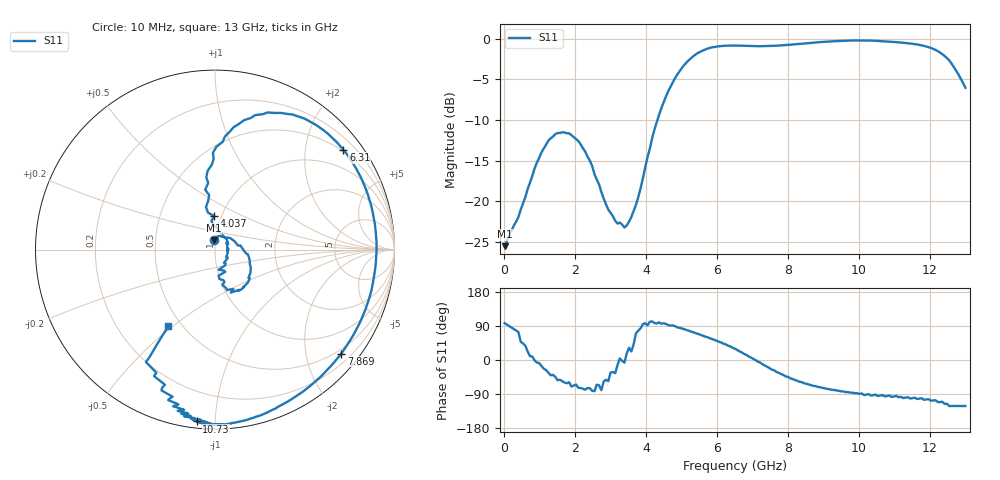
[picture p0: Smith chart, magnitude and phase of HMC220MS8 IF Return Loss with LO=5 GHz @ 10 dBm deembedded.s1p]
!Hittite Microwave Corporation
!12 Elizabeth Drive
!Chelmsford, MA 01824
!Tel: 978-250-3343
!Fax: 978-250-3373
!Device: HMC220MS8, 5-12 GHz, GaAS MMIC SMT Double-Balanced Mixer in 8-lead MSOP package
!Misc: IF Return Loss, LO = 5 GHz @ 10dBm, Room
# MHZ S MA R 50
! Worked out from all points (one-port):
!   201 points, 10 MHz to 13 GHz, reference 50 ohm
!   lowest |S11| = -25.5 dB at 10 MHz (marker M1), VSWR 1.11, Z = 49.1 + j5.17 ohm
!   |S11| at or under -10 dB: start of sweep to 4.318 GHz
!   S11 on the Smith chart (normalised r, x): 10 MHz: 0.98, +0.10; 4.037 GHz: 0.93, +0.36; 6.31 GHz: 0.46, +2.85; 7.869 GHz: 0.40, -2.74; 10.73 GHz: 0.03, -0.90; 13 GHz: 0.42, -0.48
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10  0.053 97.2
594.55  0.106 37.7
1049.2  0.2 -15.8
1633.75  0.266 -55.9
2153.35  0.224 -73.9
2932.75  0.089 -56.0
3257.5  0.074 4.2
3582.25  0.08 22.5
4036.9  0.186 91.4
4491.55  0.406 96.8
4881.25  0.603 85.8
5595.7  0.845 64.3
6310.15  0.906 37.8
6505  0.907 29.7
7154.5  0.899 -4.7
7868.95  0.912 -39.4
8128.75  0.921 -50.2
8843.2  0.95 -71.3
9752.5  0.974 -85.9
10337.05  0.974 -94.0
10661.8  0.964 -92.4
10726.75  0.963 -96.1
10856.65  0.958 -93.4
10921.6  0.957 -97.5
11376.25  0.937 -98.3
12155.65  0.853 -106.1
12545.35  0.735 -121.6
13000  0.499 -121.3
